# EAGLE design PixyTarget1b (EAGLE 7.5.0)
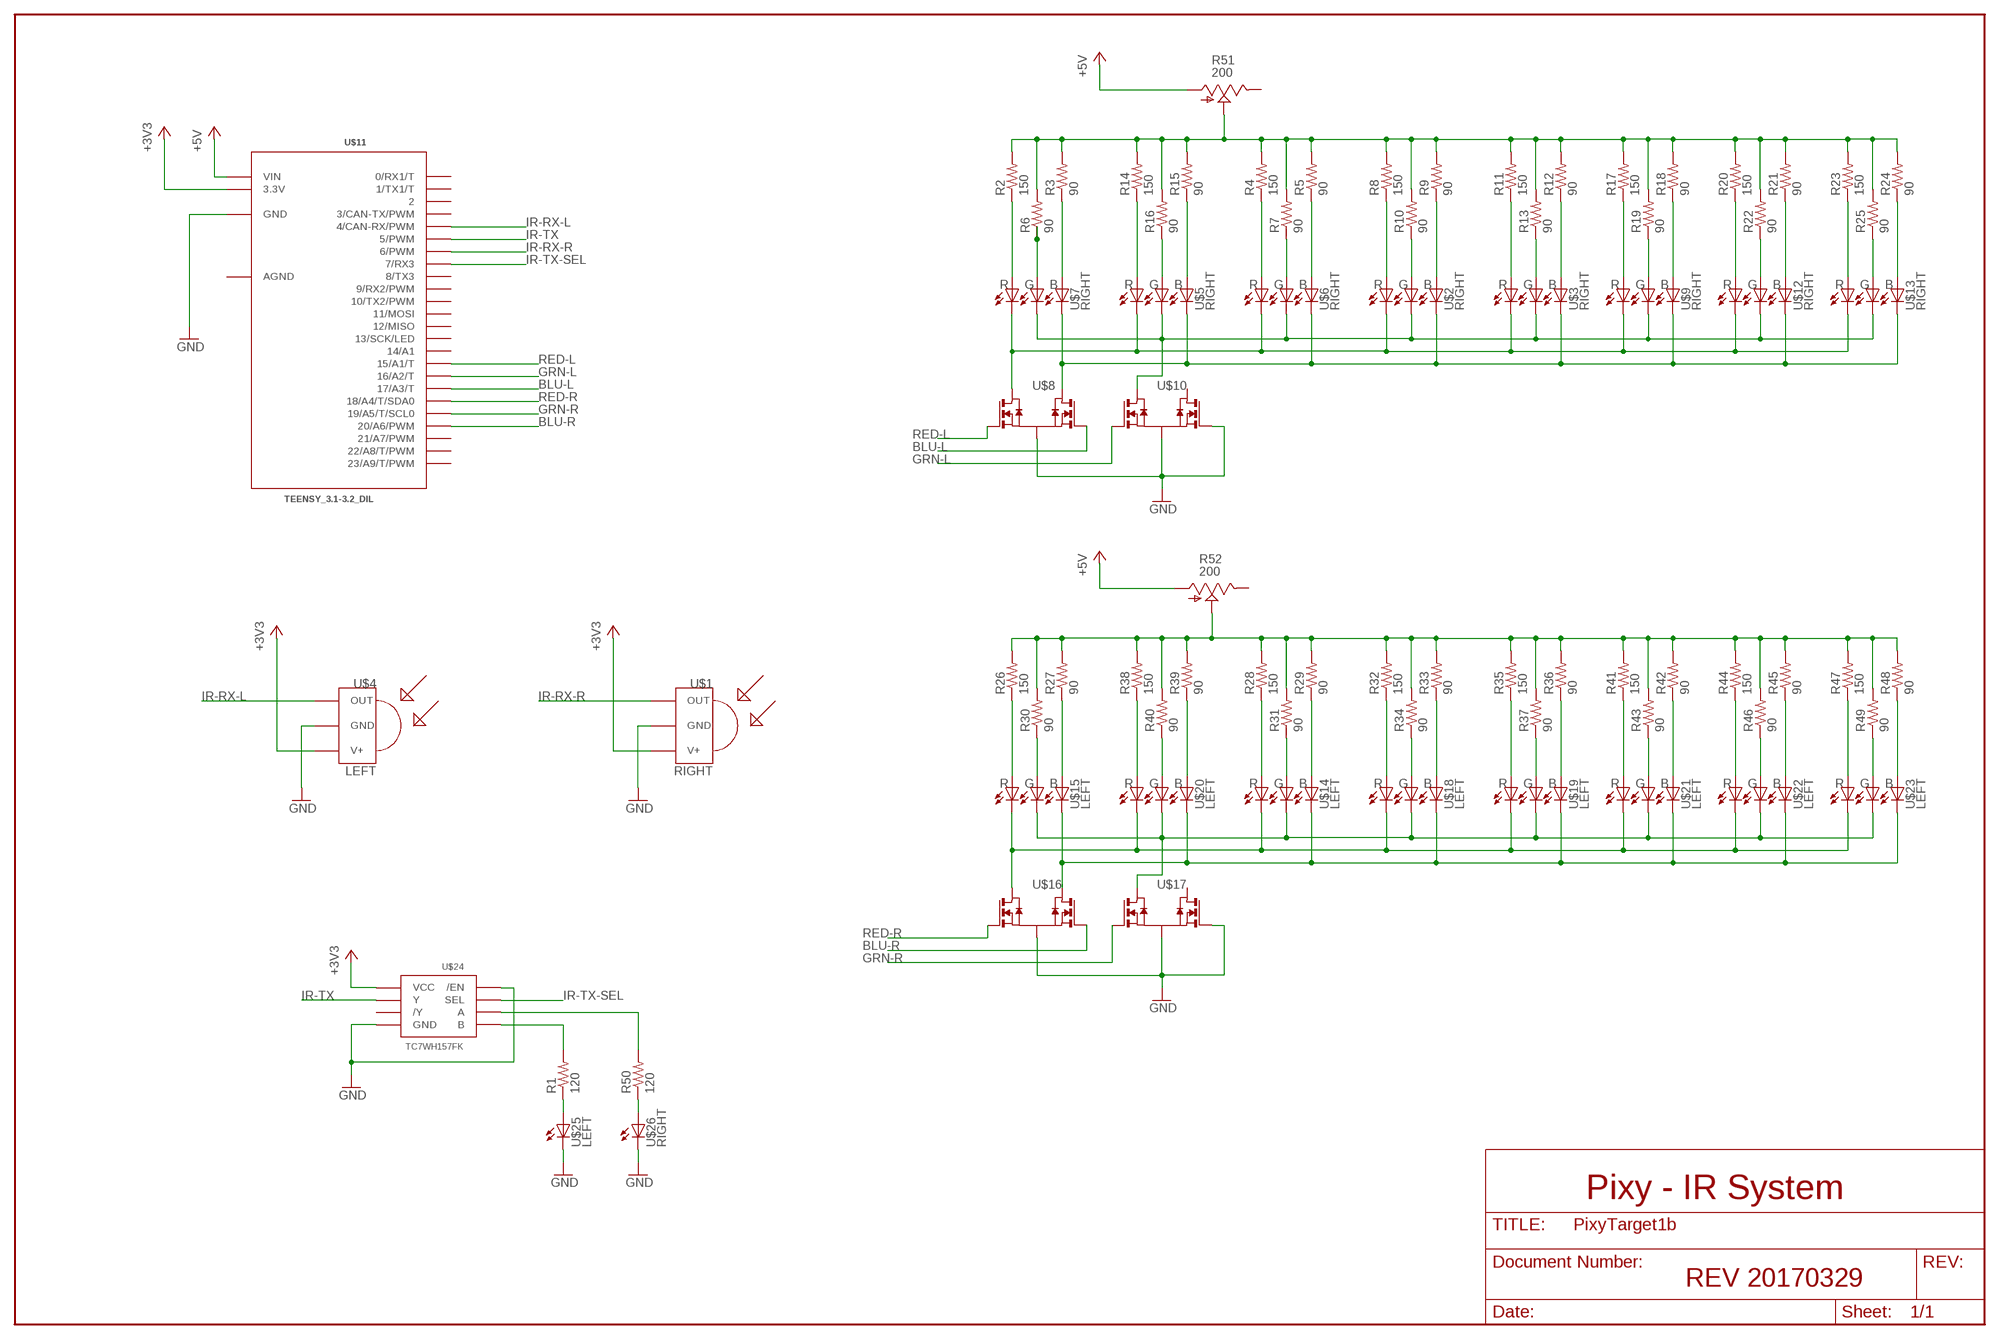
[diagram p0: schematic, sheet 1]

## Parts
R1  120  R-US_R1206  [R1206]
R2  150  R-US_R1206  [R1206]
R3  90  R-US_R1206  [R1206]
R4  150  R-US_R1206  [R1206]
R5  90  R-US_R1206  [R1206]
R6  90  R-US_R1206  [R1206]
R7  90  R-US_R1206  [R1206]
R8  150  R-US_R1206  [R1206]
R9  90  R-US_R1206  [R1206]
R10  90  R-US_R1206  [R1206]
R11  150  R-US_R1206  [R1206]
R12  90  R-US_R1206  [R1206]
R13  90  R-US_R1206  [R1206]
R14  150  R-US_R1206  [R1206]
R15  90  R-US_R1206  [R1206]
R16  90  R-US_R1206  [R1206]
R17  150  R-US_R1206  [R1206]
R18  90  R-US_R1206  [R1206]
R19  90  R-US_R1206  [R1206]
R20  150  R-US_R1206  [R1206]
R21  90  R-US_R1206  [R1206]
R22  90  R-US_R1206  [R1206]
R23  150  R-US_R1206  [R1206]
R24  90  R-US_R1206  [R1206]
R25  90  R-US_R1206  [R1206]
R26  150  R-US_R1206  [R1206]
R27  90  R-US_R1206  [R1206]
R28  150  R-US_R1206  [R1206]
R29  90  R-US_R1206  [R1206]
R30  90  R-US_R1206  [R1206]
R31  90  R-US_R1206  [R1206]
R32  150  R-US_R1206  [R1206]
R33  90  R-US_R1206  [R1206]
R34  90  R-US_R1206  [R1206]
R35  150  R-US_R1206  [R1206]
R36  90  R-US_R1206  [R1206]
R37  90  R-US_R1206  [R1206]
R38  150  R-US_R1206  [R1206]
R39  90  R-US_R1206  [R1206]
R40  90  R-US_R1206  [R1206]
R41  150  R-US_R1206  [R1206]
R42  90  R-US_R1206  [R1206]
R43  90  R-US_R1206  [R1206]
R44  150  R-US_R1206  [R1206]
R45  90  R-US_R1206  [R1206]
R46  90  R-US_R1206  [R1206]
R47  150  R-US_R1206  [R1206]
R48  90  R-US_R1206  [R1206]
R49  90  R-US_R1206  [R1206]
R50  120  R-US_R1206  [R1206]
R51  200  TRIM_US-B25P  [B25P]
R52  200  TRIM_US-B25P  [B25P]
U$1  RIGHT  TSOP3X  [TSOP18XX]
U$2  RIGHT  LED_RGB_6SMD  [6-PLCC]
U$3  RIGHT  LED_RGB_6SMD  [6-PLCC]
U$4  LEFT  TSOP3X  [TSOP18XX]
U$5  RIGHT  LED_RGB_6SMD  [6-PLCC]
U$6  RIGHT  LED_RGB_6SMD  [6-PLCC]
U$7  RIGHT  LED_RGB_6SMD  [6-PLCC]
U$8  QS5K2TR  [SOT-23-5]
U$9  RIGHT  LED_RGB_6SMD  [6-PLCC]
U$10  QS5K2TR  [SOT-23-5]
U$11  TEENSY_3.1-3.2_DIL  [TEENSY_3.0-3.2&LC_DIL]
U$12  RIGHT  LED_RGB_6SMD  [6-PLCC]
U$13  RIGHT  LED_RGB_6SMD  [6-PLCC]
U$14  LEFT  LED_RGB_6SMD  [6-PLCC]
U$15  LEFT  LED_RGB_6SMD  [6-PLCC]
U$16  QS5K2TR  [SOT-23-5]
U$17  QS5K2TR  [SOT-23-5]
U$18  LEFT  LED_RGB_6SMD  [6-PLCC]
U$19  LEFT  LED_RGB_6SMD  [6-PLCC]
U$20  LEFT  LED_RGB_6SMD  [6-PLCC]
U$21  LEFT  LED_RGB_6SMD  [6-PLCC]
U$22  LEFT  LED_RGB_6SMD  [6-PLCC]
U$23  LEFT  LED_RGB_6SMD  [6-PLCC]
U$24  TC7WH157FK  [SSOP8-P-0.65]
U$25  LEFT  LED5MM  [LED5MM]
U$26  RIGHT  LED5MM  [LED5MM]

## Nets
+3V3: U$1.VCC(V+) U$4.VCC(V+) U$11.3.3V U$24.P$8(VCC)
+5V: R51.A R52.A U$11.VIN
BLU-L: U$8.3(G2) U$11.17/A3(17/A3/T)
BLU-R: U$11.20/A6(20/A6/PWM) U$16.3(G2)
GND [ground]: U$1.GND U$4.GND U$8.2(S) U$10.2(S) U$10.3(G2) U$11.GND U$16.2(S) U$17.2(S) U$17.3(G2) U$24.P$4(GND) U$24.P$7(/EN) U$25.K(C) U$26.K(C)
GRN-L: U$10.1(G1) U$11.16/A2(16/A2/T)
GRN-R: U$11.19/A5(19/A5/T/SCL0) U$17.1(G1)
IR-RX-L: U$4.OUT U$11.4(4/CAN-RX/PWM)
IR-RX-R: U$1.OUT U$11.6(6/PWM)
IR-TX: U$11.5(5/PWM) U$24.P$5(Y)
IR-TX-SEL: U$11.7(7/RX3) U$24.P$6(SEL)
N$1: R8.1 U$2.P$1(A1)
N$2: R9.1 U$2.P$3(A3)
N$3: R2.1 U$7.P$1(A1)
N$4: R3.1 U$7.P$3(A3)
N$5: R6.1 U$7.P$2(A2)
N$6: R26.1 U$15.P$1(A1)
N$7: R10.1 U$2.P$2(A2)
N$8: U$2.P$6(C1) U$3.P$6(C1) U$5.P$6(C1) U$6.P$6(C1) U$7.P$6(C1) U$8.5(D1) U$9.P$6(C1) U$12.P$6(C1) U$13.P$6(C1)
N$9: U$2.P$4(C3) U$3.P$4(C3) U$5.P$4(C3) U$6.P$4(C3) U$7.P$4(C3) U$8.4(D2) U$9.P$4(C3) U$12.P$4(C3) U$13.P$4(C3)
N$10: R1.1 U$25.A
N$11: R20.1 U$12.P$1(A1)
N$12: R11.1 U$3.P$1(A1)
N$13: R12.1 U$3.P$3(A3)
N$14: R13.1 U$3.P$2(A2)
N$15: R17.1 U$9.P$1(A1)
N$16: R18.1 U$9.P$3(A3)
N$17: R14.1 U$5.P$1(A1)
N$18: R15.1 U$5.P$3(A3)
N$19: R19.1 U$9.P$2(A2)
N$20: R21.1 U$12.P$3(A3)
N$21: R16.1 U$5.P$2(A2)
N$22: U$2.P$5(C2) U$3.P$5(C2) U$5.P$5(C2) U$6.P$5(C2) U$7.P$5(C2) U$9.P$5(C2) U$10.5(D1) U$12.P$5(C2) U$13.P$5(C2)
N$23: R22.1 U$12.P$2(A2)
N$24: R27.1 U$15.P$3(A3)
N$25: R4.1 U$6.P$1(A1)
N$26: R5.1 U$6.P$3(A3)
N$27: R30.1 U$15.P$2(A2)
N$28: R7.1 U$6.P$2(A2)
N$29: R23.1 U$13.P$1(A1)
N$30: R24.1 U$13.P$3(A3)
N$31: R25.1 U$13.P$2(A2)
N$32: R28.1 U$14.P$1(A1)
N$33: R29.1 U$14.P$3(A3)
N$34: R31.1 U$14.P$2(A2)
N$35: R32.1 U$18.P$1(A1)
N$36: R33.1 U$18.P$3(A3)
N$37: R34.1 U$18.P$2(A2)
N$38: U$14.P$6(C1) U$15.P$6(C1) U$16.5(D1) U$18.P$6(C1) U$19.P$6(C1) U$20.P$6(C1) U$21.P$6(C1) U$22.P$6(C1) U$23.P$6(C1)
N$39: R35.1 U$19.P$1(A1)
N$40: R36.1 U$19.P$3(A3)
N$41: R37.1 U$19.P$2(A2)
N$42: U$14.P$4(C3) U$15.P$4(C3) U$16.4(D2) U$18.P$4(C3) U$19.P$4(C3) U$20.P$4(C3) U$21.P$4(C3) U$22.P$4(C3) U$23.P$4(C3)
N$43: R38.1 U$20.P$1(A1)
N$44: R39.1 U$20.P$3(A3)
N$45: R40.1 U$20.P$2(A2)
N$46: U$14.P$5(C2) U$15.P$5(C2) U$17.5(D1) U$18.P$5(C2) U$19.P$5(C2) U$20.P$5(C2) U$21.P$5(C2) U$22.P$5(C2) U$23.P$5(C2)
N$47: R41.1 U$21.P$1(A1)
N$48: R42.1 U$21.P$3(A3)
N$49: R43.1 U$21.P$2(A2)
N$50: R44.1 U$22.P$1(A1)
N$51: R45.1 U$22.P$3(A3)
N$52: R46.1 U$22.P$2(A2)
N$53: R47.1 U$23.P$1(A1)
N$54: R48.1 U$23.P$3(A3)
N$55: R49.1 U$23.P$2(A2)
N$56: R50.2 U$24.P$1(A)
N$57: R50.1 U$26.A
N$58: R1.2 U$24.P$2(B)
N$59: R2.2 R3.2 R4.2 R5.2 R6.2 R7.2 R8.2 R9.2 R10.2 R11.2 R12.2 R13.2 R14.2 R15.2 R16.2 R17.2 R18.2 R19.2 R20.2 R21.2 R22.2 R23.2 R24.2 R25.2 R51.S
N$60: R26.2 R27.2 R28.2 R29.2 R30.2 R31.2 R32.2 R33.2 R34.2 R35.2 R36.2 R37.2 R38.2 R39.2 R40.2 R41.2 R42.2 R43.2 R44.2 R45.2 R46.2 R47.2 R48.2 R49.2 R52.S
RED-L: U$8.1(G1) U$11.15/A1(15/A1/T)
RED-R: U$11.18/A4(18/A4/T/SDA0) U$16.1(G1)
Unconnected: R51.E R52.E U$10.4(D2) U$11.0(0/RX1/T) U$11.1(1/TX1/T) U$11.2 U$11.3(3/CAN-TX/PWM) U$11.8(8/TX3) U$11.9(9/RX2/PWM) U$11.10(10/TX2/PWM) U$11.11(11/MOSI) U$11.12(12/MISO) U$11.13(13/SCK/LED) U$11.14/A0(14/A1) U$11.21/A7(21/A7/PWM) U$11.22/A8(22/A8/T/PWM) U$11.23/A9(23/A9/T/PWM) U$17.4(D2) U$24.P$3(/Y)

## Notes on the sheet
- Pixy - IR System
- REV 20170329

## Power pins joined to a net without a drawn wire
GND: U$11.AGND

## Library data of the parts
R1-R50 = resistor:R-US_: RESISTOR, American symbol
R51 R52 = pot:TRIM_US-: POTENTIOMETER
U$1 U$4 = _Loper:TSOP3X: IR Receiver and Demodulator
U$2 U$3 U$5-U$7 U$9 U$12-U$15 U$18-U$23 = _Loper:LED_RGB_6SMD
U$8 U$10 U$16 U$17 = _Loper:QS5K2TR: MOSFET 2N-CH
U$11 = Teensy_3_and_LC_Series_Boards_v1.4:TEENSY_3.1-3.2_DIL: Teensy 3.1 or 3.2 in a DIL Layout.
U$24 = _Loper:TC7WH157FK: multiplexer 1x 2:1
U$25 U$26 = led:LED: LED

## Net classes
0 default: width 0.406 mm
1 ground: width 0.61 mm

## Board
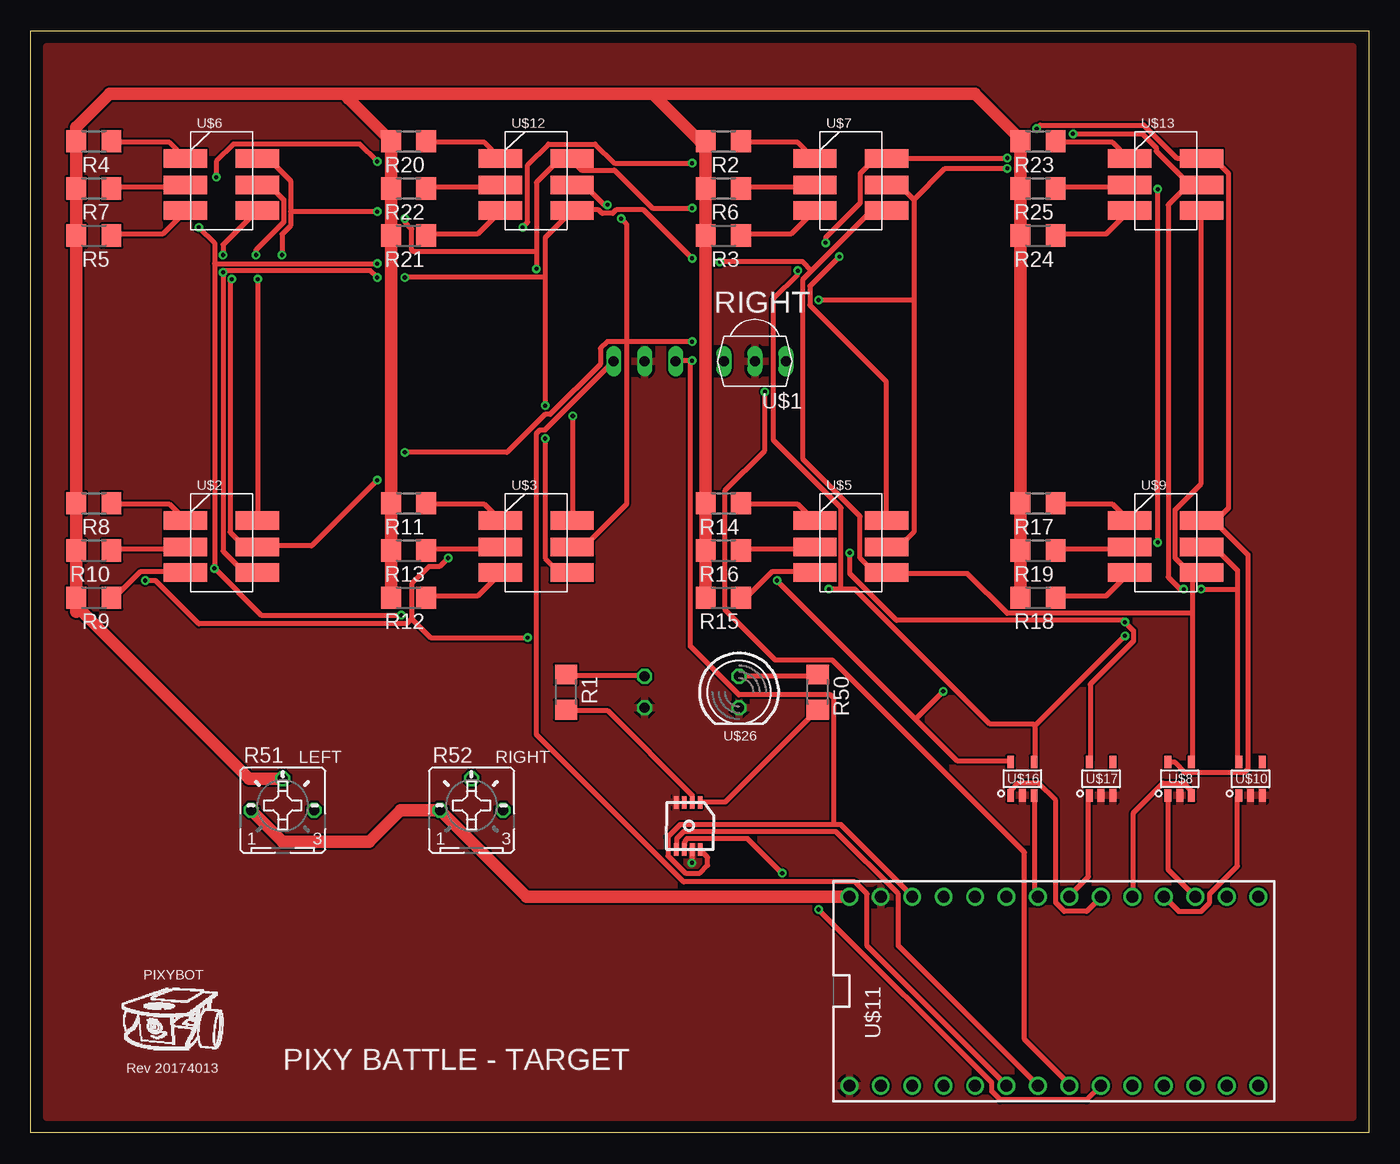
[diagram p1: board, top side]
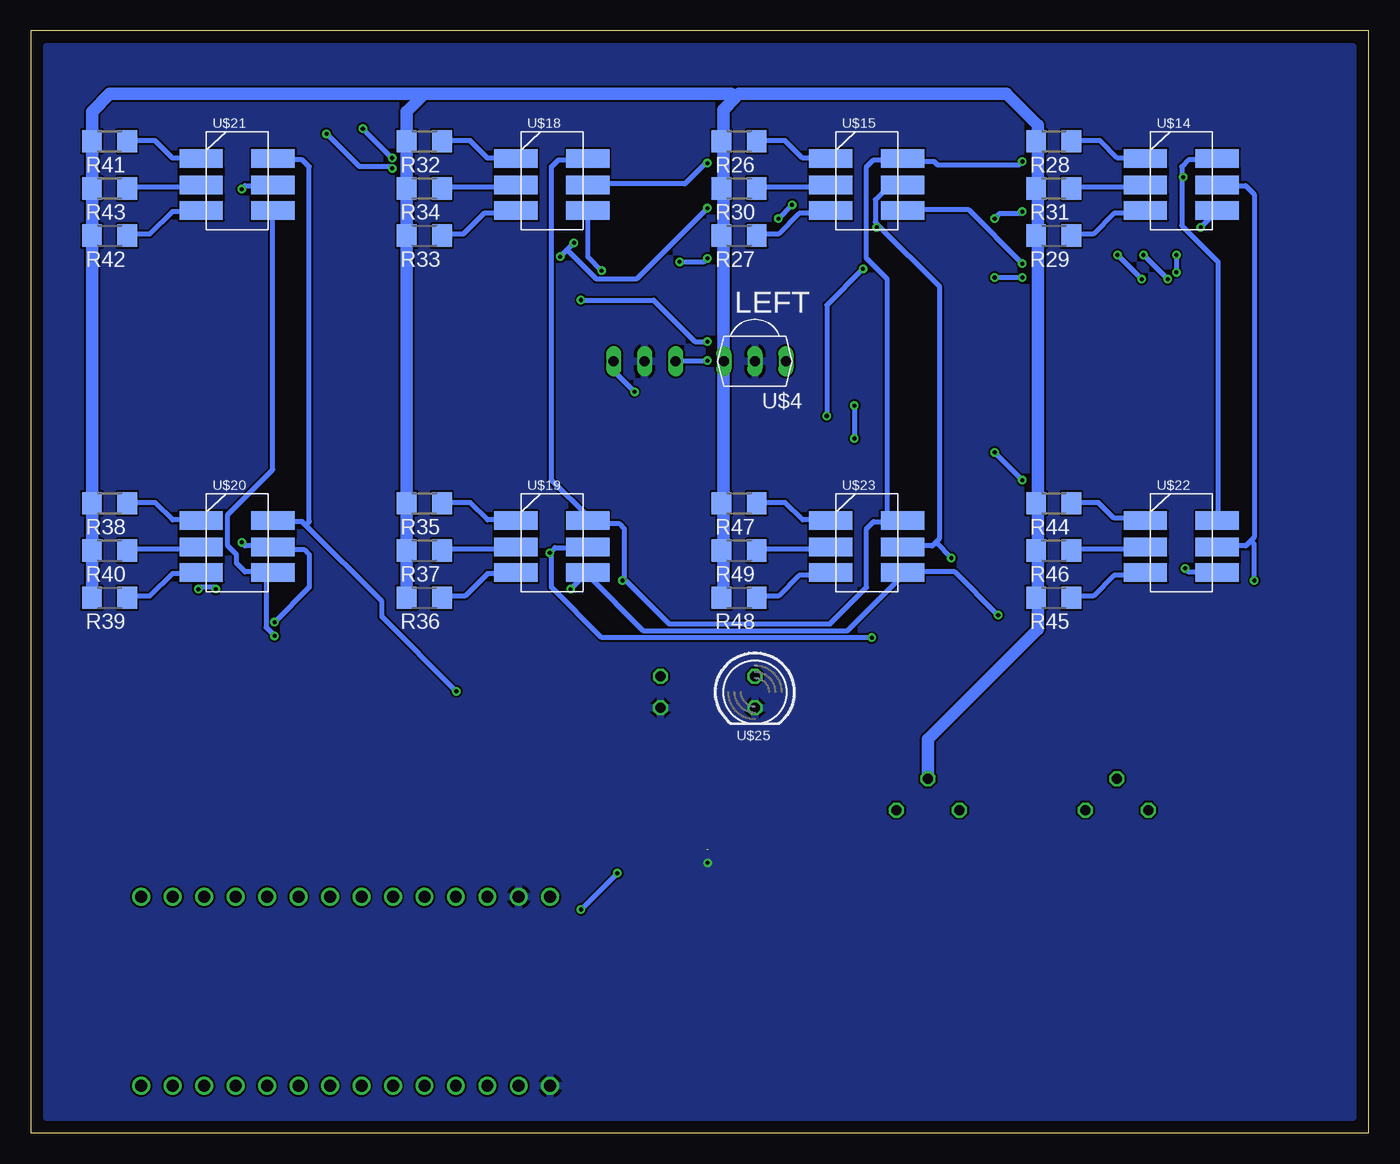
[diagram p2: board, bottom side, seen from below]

Size 107.95 x 88.9 mm. Coordinates in mm from the lower left corner, seen from the top.
Outline: 0,0 0,88.9 107.95,88.9 107.95,0 0,0
Copper layers (1*16): Top 0.0356mm / dielectric 1.5011mm / Bottom 0.0356mm
Design rules "oshpark-2layer": minimum track width 6mil, minimum drill 13mil, track to track 6mil, track to pad 6mil, pad to pad 6mil, via to via 6mil, smd to smd 6mil, copper to edge 15mil, drill to drill 6mil, minimum pad ring 7mil, minimum via ring 7mil, stop-mask expansion 2.5mil, vias tented up to drill 0mil, thermal gap 10mil

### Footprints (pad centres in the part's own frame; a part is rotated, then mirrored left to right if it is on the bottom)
R1206 = smd 1.6 x 1.803: 1 -1.422,0; 2 1.422,0
B25P = drill 0.813 octagon: A -2.54,0; E 2.54,0; S 0,2.54
TSOP18XX = drill 0.813 long: GND -0.001,-0.027; OUT -2.501,-0.027; VCC 2.499,-0.027
6-PLCC = smd 3.5 x 1.5: P$1 -2.77,2.41; P$2 -2.77,0.29; P$3 -2.77,-1.78; P$4 3.03,-1.78; P$5 3.03,0.29; P$6 3.03,2.41
SOT-23-5 = smd 1 x 0.55: 1 -1.35,0.95; 2 -1.35,0; 3 -1.35,-0.95; 4 1.35,-0.95; 5 1.35,0.95
TEENSY_3.0-3.2&LC_DIL = drill 0.965: 0 -7.62,13.97; 1 -7.62,11.43; 2 -7.62,8.89; 3 -7.62,6.35; 3.3V 7.62,11.43; 4 -7.62,3.81; 5 -7.62,1.27; 6 -7.62,-1.27; 7 -7.62,-3.81; 8 -7.62,-6.35; 9 -7.62,-8.89; 10 -7.62,-11.43; 11 -7.62,-13.97; 12 -7.62,-16.51; 13 7.62,-16.51; 14/A0 7.62,-13.97; 15/A1 7.62,-11.43; 16/A2 7.62,-8.89; 17/A3 7.62,-6.35; 18/A4 7.62,-3.81; 19/A5 7.62,-1.27; 20/A6 7.62,1.27; 21/A7 7.62,3.81; 22/A8 7.62,6.35; 23/A9 7.62,8.89; AGND 7.62,13.97; GND -7.62,16.51; VIN 7.62,16.51
SSOP8-P-0.65 = smd 1 x 0.35: P$1 0,1.95; P$2 0,1.3; P$3 0,0.65; P$4 0,0; P$5 3.8,0; P$6 3.8,0.65; P$7 3.8,1.3; P$8 3.8,1.95
LED5MM = drill 0.813 octagon: A -1.27,0; K 1.27,0

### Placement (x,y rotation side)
R1  43.18,35.56 270 top
R2  55.88,80.01 180 top
R3  55.88,72.39 180 top
R4  5.08,80.01 180 top
R5  5.08,72.39 180 top
R6  55.88,76.2 180 top
R7  5.08,76.2 180 top
R8  5.08,50.8 180 top
R9  5.08,43.18 180 top
R10  5.08,46.99 180 top
R11  30.48,50.8 180 top
R12  30.48,43.18 180 top
R13  30.48,46.99 180 top
R14  55.88,50.8 180 top
R15  55.88,43.18 180 top
R16  55.88,46.99 180 top
R17  81.28,50.8 180 top
R18  81.28,43.18 180 top
R19  81.28,46.99 180 top
R20  30.48,80.01 180 top
R21  30.48,72.39 180 top
R22  30.48,76.2 180 top
R23  81.28,80.01 180 top
R24  81.28,72.39 180 top
R25  81.28,76.2 180 top
R26  50.8,80.01 180 bottom
R27  50.8,72.39 180 bottom
R28  25.4,80.01 180 bottom
R29  25.4,72.39 180 bottom
R30  50.8,76.2 180 bottom
R31  25.4,76.2 180 bottom
R32  76.2,80.01 180 bottom
R33  76.2,72.39 180 bottom
R34  76.2,76.2 180 bottom
R35  76.2,50.8 180 bottom
R36  76.2,43.18 180 bottom
R37  76.2,46.99 180 bottom
R38  101.6,50.8 180 bottom
R39  101.6,43.18 180 bottom
R40  101.6,46.99 180 bottom
R41  101.6,80.01 180 bottom
R42  101.6,72.39 180 bottom
R43  101.6,76.2 180 bottom
R44  25.4,50.8 180 bottom
R45  25.4,43.18 180 bottom
R46  25.4,46.99 180 bottom
R47  50.8,50.8 180 bottom
R48  50.8,43.18 180 bottom
R49  50.8,46.99 180 bottom
R50  63.5,35.56 270 top
R51  20.32,26.04 0 top
R52  35.56,26.04 0 top
U$1  58.42,62.23 180 top
U$2  15.24,46.99 0 top
U$3  40.64,46.99 0 top
U$4  49.53,62.23 180 bottom
U$5  66.04,46.99 0 top
U$6  15.24,76.2 0 top
U$7  66.04,76.2 0 top
U$8  92.71,28.57 90 top
U$9  91.44,46.99 0 top
U$10  98.42,28.57 90 top
U$11  82.55,11.43 90 top
U$12  40.64,76.2 0 top
U$13  91.44,76.2 0 top
U$14  15.24,76.2 0 bottom
U$15  40.64,76.2 0 bottom
U$16  80.01,28.57 90 top
U$17  86.36,28.57 90 top
U$18  66.04,76.2 0 bottom
U$19  66.04,46.99 0 bottom
U$20  91.44,46.99 0 bottom
U$21  91.44,76.2 0 bottom
U$22  15.24,46.99 0 bottom
U$23  40.64,46.99 0 bottom
U$24  52.07,26.67 270 top
U$25  49.53,35.56 270 bottom
U$26  57.15,35.56 270 top

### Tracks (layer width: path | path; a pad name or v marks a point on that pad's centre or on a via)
+3V3  (via drill 0.33)
  Top 0.406: U$4.VCC 52.11,62.31 v53.37,62.31 53.23,62.17 53.23,39.26 57.14,35.34 64.54,35.34 64.82,35.06 64.82,24.87 | 64.82,24.87 65.38,24.87 71.11,19.14 U$11.3.3V | 64.82,24.87 52.39,24.87 51.41,23.89 51.41,22.35 52.81,20.95 53.98,20.95 54.61,21.59 54.61,22.23 54.02,22.82 U$24.P$8
  Bottom 0.406: v53.37,62.31 55.88,62.31 U$1.VCC
+5V
  Top 1.016: U$11.VIN 40.01,19.05 R52.A 29.84,26.04 27.3,23.5 20.32,23.5 R51.A
BLU-L
  Top 0.406: U$8.3 93.6,27.24 93.6,27.66 93.04,28.22 91.36,28.22 88.99,25.84 88.99,19.14 U$11.17/A3
BLU-R
  Top 0.406: U$16.3 81.03,27.1 81.03,19.28 81.17,19.14 U$11.20/A6
GND  (via drill 0.33)  (1 unrouted)
  Top 0.406: 53.34,22.84 v53.34,21.79
  pour Bottom: 1.27,1.27 106.68,1.27 106.68,87.63 1.27,87.63
  pour Top: 1.27,1.27 106.68,1.27 106.68,87.63 1.27,87.63
GRN-L
  Top 0.406: U$10.1 97.37,27.1 97.37,21.51 95.14,19.28 95.14,18.58 94.44,17.88 92.62,17.88 91.5,19 U$11.16/A2
GRN-R
  Top 0.406: U$17.1 85.36,27.1 85.36,20.68 83.82,19.14 U$11.19/A5
IR-RX-L
  Top 0.406: U$4.OUT 46.94,62.17 41.49,56.72 41.07,56.72 40.79,56.44 40.79,32.13 52.67,20.26 66.5,20.26 67.47,19.28 67.47,15.09 78.65,3.91 U$11.4
IR-RX-R  (via drill 0.33)
  Top 0.406: v59.23,59.79 59.23,55.04 56.02,51.83 56.02,42.19 60.07,38.14 64.68,38.14 80.19,22.63 80.19,7.54 83.82,3.91 U$11.6
  Bottom 0.406: v59.23,59.79 60.91,61.47 60.91,62.17 U$1.OUT
IR-TX
  Top 0.406: U$24.P$5 52.11,22.91 52.11,23.75 52.67,24.31 64.96,24.31 69.99,19.28 69.99,15.09 81.17,3.91 U$11.5
IR-TX-SEL  (via drill 0.33)
  Top 0.406: v60.63,20.95 57.84,23.75 52.95,23.75 52.81,23.61 52.73,23.42 U$24.P$6 | v63.56,18.02 77.53,4.05 77.53,3.35 78.23,2.65 85.22,2.65 86.33,3.77 U$11.7
  Bottom 0.406: v63.56,18.02 v60.63,20.95
N$1
  Top 0.406: R8.1 6.57,50.71 11.18,50.71 12.43,49.45 U$2.P$1
N$2
  Top 0.406: R9.1 6.57,43.31 6.84,43.31 8.8,45.26 12.43,45.26 U$2.P$3
N$3
  Top 0.406: R2.1 57.42,79.91 61.89,79.91 63.14,78.65 U$7.P$1
N$4
  Top 0.406: R3.1 57.42,72.5 61.33,72.5 63.14,74.32 U$7.P$3
N$5
  Top 0.406: R6.1 57.42,76.28 63.01,76.28 63.14,76.42 U$7.P$2
N$6
  Bottom 0.406: R26.1 49.31,80.05 47.08,80.05 45.68,78.65 43.45,78.65 U$15.P$1
N$7
  Top 0.406: R10.1 6.57,47.08 12.29,47.08 12.43,47.22 U$2.P$2
N$8  (via drill 0.33)
  Top 0.406: U$8.5 91.78,29.9 92.34,29.9 93.18,29.06 97.93,29.06 98.21,29.34 98.21,46.66 95.56,49.31 94.58,49.31 U$9.P$6 95.69,49.45 96.67,50.43 96.67,77.39 95.56,78.51 94.58,78.51 U$13.P$6 94.3,78.65 92.48,78.65 89.83,81.31 81.44,81.31 v81.17,81.03 | v65.24,70.69 62.87,68.31 62.87,66.78 69.01,60.63 69.01,49.45 U$5.P$6 | v64.12,71.81 64.12,72.22 66.92,75.02 66.92,77.39 68.03,78.51 69.01,78.51 U$7.P$6 69.15,78.65 v78.79,78.65 | v18.3,68.87 18.3,49.45 U$2.P$6 | v20.26,70.83 20.26,72.5 20.95,73.2 20.95,74.32 | 20.95,74.32 20.95,76.83 19.28,78.51 18.3,78.51 U$6.P$6 | v43.73,57.84 43.73,49.45 U$3.P$6 | 40.79,71.11 40.79,76.69 42.61,78.51 43.59,78.51 U$12.P$6 43.73,78.37 44.42,77.67 47.08,77.67 50.15,74.6 v53.37,74.6 | 40.79,71.11 v40.79,69.71 | v27.94,74.32 20.95,74.32 | v30.18,73.76 30.18,73.48 30.73,72.92 30.73,71.25 30.87,71.11 40.79,71.11
  Bottom 0.406: v64.12,71.81 64.68,71.25 | 64.68,71.25 v65.24,70.69 | v20.26,70.83 v18.3,68.87 | v43.73,57.84 43.73,66.78 v40.79,69.71 | v27.94,74.32 28.08,74.18 29.76,74.18 v30.18,73.76 | 64.68,71.25 62.31,68.87 59.09,68.87 v53.37,74.6 | v78.79,78.65 v81.17,81.03
N$9  (via drill 0.33)
  Top 0.406: v15.51,70.83 15.51,71.67 18.16,74.32 U$6.P$4 | U$2.P$4 18.16,45.26 17.18,45.26 15.51,46.94 v15.51,69.43 15.65,69.57 27.38,69.57 v27.94,69.01 | v41.49,56.02 41.49,46.38 42.61,45.26 43.59,45.26 U$3.P$4 | 41.49,69.01 41.49,72.22 43.59,74.32 U$12.P$4 43.87,74.46 45.82,74.46 46.1,74.18 46.94,74.18 47.22,74.46 49.45,74.46 v53.37,70.55 | 41.49,69.01 v41.49,58.67 | 93.74,41.91 93.74,44.42 94.44,45.12 U$9.P$4 93.88,44.84 92.34,46.38 92.34,50.29 94.44,52.39 94.44,74.32 U$13.P$4 | 93.74,41.91 93.74,30.04 U$8.4 | 93.74,41.91 78.79,41.91 75.58,45.12 69.15,45.12 U$5.P$4 68.87,45.26 68.03,45.26 66.92,46.38 66.92,49.73 62.31,54.34 62.31,68.87 63.01,69.57 | 63.01,69.57 67.75,74.32 69.01,74.32 U$7.P$4 | v55.6,70.27 62.31,70.27 63.01,69.57 | 41.49,69.01 v30.18,69.01
  Bottom 0.406: v15.51,70.83 v15.51,69.43 | v41.49,58.67 v41.49,56.02 | v53.37,70.55 53.65,70.27 v55.6,70.27 | v30.18,69.01 v27.94,69.01
N$10
  Top 0.406: R1.1 43.31,36.88 49.45,36.88 U$25.A
N$11
  Top 0.406: R20.1 31.99,79.91 36.6,79.91 37.86,78.65 U$12.P$1
N$12
  Top 0.406: R11.1 31.99,50.71 36.6,50.71 37.86,49.45 U$3.P$1
N$13
  Top 0.406: R12.1 31.99,43.31 36.04,43.31 37.86,45.12 U$3.P$3
N$14
  Top 0.406: R13.1 31.99,47.08 37.72,47.08 37.86,47.22 U$3.P$2
N$15
  Top 0.406: R17.1 82.7,50.71 87.31,50.71 88.57,49.45 U$9.P$1
N$16
  Top 0.406: R18.1 82.7,43.31 86.75,43.31 88.57,45.12 U$9.P$3
N$17
  Top 0.406: R14.1 57.42,50.71 61.89,50.71 63.14,49.45 U$5.P$1
N$18
  Top 0.406: R15.1 57.42,43.31 57.84,43.31 59.79,45.26 63.14,45.26 U$5.P$3
N$19
  Top 0.406: R19.1 82.7,47.08 88.43,47.08 88.57,47.22 U$9.P$2
N$20
  Top 0.406: R21.1 31.99,72.5 36.04,72.5 37.86,74.32 U$12.P$3
N$21
  Top 0.406: R16.1 57.42,47.08 63.01,47.08 63.14,47.22 U$5.P$2
N$22  (via drill 0.33)
  Top 0.406: v16.2,68.87 16.07,68.73 16.07,48.48 17.18,47.36 18.16,47.36 U$2.P$5 18.44,47.36 22.63,47.36 v27.94,52.67 | v18.16,70.83 18.16,71.25 20.4,73.48 20.4,75.3 19.28,76.42 18.3,76.42 U$6.P$5 | 48.06,63.84 48.06,73.34 v47.64,73.76 | 48.06,63.84 48.06,50.71 44.7,47.36 43.73,47.36 U$3.P$5 | v46.52,74.88 46.24,74.88 44.7,76.42 43.73,76.42 U$12.P$5 | v30.18,54.9 38.42,54.9 41.49,57.98 41.91,57.98 45.96,62.03 45.96,63.28 46.52,63.84 48.06,63.84 | 97.37,43.87 97.37,45.4 95.56,47.22 94.58,47.22 U$9.P$5 | 97.37,43.87 97.37,30.04 U$10.5 | 71.25,75.3 71.25,67.2 | 71.25,67.2 71.25,48.48 70.13,47.36 69.15,47.36 U$5.P$5 | 71.25,75.3 70.13,76.42 69.15,76.42 U$7.P$5 | v84.1,80.61 89.69,80.61 90.81,79.49 90.81,79.21 93.46,76.56 94.44,76.56 U$13.P$5 93.32,76.42 91.78,74.88 91.78,44.84 92.76,43.87 v93.04,43.87 | v78.79,77.81 73.76,77.81 71.25,75.3 | v94.44,43.87 97.37,43.87 | v53.37,63.84 48.06,63.84 | 71.25,67.2 v63.56,67.2
  Bottom 0.406: v18.16,70.83 v16.2,68.87 | v46.52,74.88 v47.64,73.76 | v30.18,54.9 v27.94,52.67 | v84.1,80.61 81.44,77.95 78.93,77.95 v78.79,77.81 | v94.44,43.87 94.3,44.01 93.18,44.01 v93.04,43.87 | v53.37,63.84 54.34,63.84 57.7,67.2 v63.56,67.2
N$23
  Top 0.406: R22.1 31.99,76.28 37.72,76.28 37.86,76.42 U$12.P$2
N$24
  Bottom 0.406: R27.1 49.31,72.5 47.64,72.5 45.96,74.18 43.59,74.18 43.45,74.32 U$15.P$3
N$25
  Top 0.406: R4.1 6.57,79.91 11.18,79.91 12.43,78.65 U$6.P$1
N$26
  Top 0.406: R5.1 6.57,72.5 10.62,72.5 12.43,74.32 U$6.P$3
N$27
  Bottom 0.406: R30.1 49.31,76.28 43.59,76.28 43.45,76.42 U$15.P$2
N$28
  Top 0.406: R7.1 6.57,76.28 12.29,76.28 12.43,76.42 U$6.P$2
N$29
  Top 0.406: R23.1 82.7,79.91 87.31,79.91 88.57,78.65 U$13.P$1
N$30
  Top 0.406: R24.1 82.7,72.5 86.75,72.5 88.57,74.32 U$13.P$3
N$31
  Top 0.406: R25.1 82.7,76.28 88.43,76.28 88.57,76.42 U$13.P$2
N$32
  Bottom 0.406: R28.1 23.89,80.05 21.65,80.05 20.26,78.65 18.02,78.65 U$14.P$1
N$33
  Bottom 0.406: R29.1 23.89,72.5 22.21,72.5 20.54,74.18 18.16,74.18 18.02,74.32 U$14.P$3
N$34
  Bottom 0.406: R31.1 23.89,76.28 18.16,76.28 18.02,76.42 U$14.P$2
N$35
  Bottom 0.406: R32.1 74.74,80.05 72.5,80.05 71.11,78.65 68.87,78.65 U$18.P$1
N$36
  Bottom 0.406: R33.1 74.74,72.5 73.06,72.5 71.39,74.18 69.01,74.18 68.87,74.32 U$18.P$3
N$37
  Bottom 0.406: R34.1 74.74,76.28 69.01,76.28 68.87,76.42 U$18.P$2
N$38  (via drill 0.33)
  Top 0.406: v60.21,44.56 71.39,33.39 | 71.39,33.39 74.74,30.04 78.93,30.04 U$16.5 | 71.39,33.39 v73.62,35.62 | v14.95,77.11 14.95,78.37 16.34,79.77 26.54,79.77 v27.94,78.37
  Bottom 0.406: 15.09,77.11 15.09,77.95 14.53,78.51 12.29,78.51 U$14.P$6 | 15.09,77.11 15.09,73.2 12.15,70.27 12.15,49.45 U$22.P$6 | 85.78,49.03 79.63,42.89 79.63,41.63 v73.62,35.62 | 85.78,49.03 86.06,49.31 88.29,49.31 U$20.P$6 | U$18.P$6 63.14,78.51 65.38,78.51 65.94,77.95 65.94,52.67 63.01,49.73 63.01,49.59 U$19.P$6 63.01,49.31 62.87,49.17 60.49,49.17 60.07,48.76 60.07,44.7 v60.21,44.56 59.93,44.56 56.44,41.07 43.45,41.07 40.51,44.01 40.51,48.76 39.95,49.31 37.72,49.31 U$23.P$6 38.84,49.45 38.84,68.87 40.51,70.55 40.51,77.95 39.95,78.51 37.72,78.51 U$15.P$6 37.58,78.37 35.06,78.37 34.78,78.09 28.22,78.09 v27.94,78.37 | U$21.P$6 88.29,78.51 86.06,78.51 85.5,77.95 85.5,49.31 85.78,49.03 | v14.95,77.11 15.09,77.11
N$39
  Bottom 0.406: R35.1 74.74,50.85 72.5,50.85 71.11,49.45 68.87,49.45 U$19.P$1
N$40
  Bottom 0.406: R36.1 74.74,43.31 72.92,43.31 71.11,45.12 68.87,45.12 U$19.P$3
N$41
  Bottom 0.406: R37.1 74.74,47.08 69.01,47.08 68.87,47.22 U$19.P$2
N$42  (via drill 0.33)
  Top 0.406: 14.81,70.13 14.81,71.81 v13.55,73.06 | 14.81,70.13 v14.81,45.54 18.58,41.77 v29.9,41.77 | 14.81,70.13 v27.94,70.13 | 81.03,32.83 81.03,30.04 U$16.4 | v88.29,40.09 81.03,32.83 | 65.38,43.87 66.5,43.87 77.39,32.97 80.89,32.97 81.03,32.83 | 65.38,43.87 v64.4,43.87 | v61.89,69.57 61.89,69.29 59.93,67.33 59.93,55.88 65.38,50.43 65.38,43.87
  Bottom 0.406: v14.81,45.54 14.53,45.26 12.29,45.26 U$22.P$4 | v13.55,73.06 12.29,74.32 U$14.P$4 | v29.9,41.77 33.39,45.26 37.58,45.26 U$23.P$4 37.72,45.12 37.72,44.84 42.05,40.51 58.53,40.51 63.01,44.98 U$19.P$4 63.14,45.12 v64.4,43.87 | v27.94,70.13 32.27,74.46 37.58,74.46 U$15.P$4 | v88.29,40.09 88.99,40.79 88.99,44.56 88.43,45.12 U$20.P$4 89.13,44.7 89.69,45.26 90.67,45.26 91.36,45.96 91.36,46.66 92.06,47.36 92.06,49.87 88.43,53.51 88.43,74.32 U$21.P$4 | v61.89,69.57 63.01,70.69 63.01,74.32 U$18.P$4
N$43
  Bottom 0.406: R38.1 100.17,50.85 97.93,50.85 96.53,49.45 94.3,49.45 U$20.P$1
N$44
  Bottom 0.406: R39.1 100.17,43.31 98.35,43.31 96.53,45.12 94.3,45.12 U$20.P$3
N$45
  Bottom 0.406: R40.1 100.17,47.08 94.44,47.08 94.3,47.22 U$20.P$2
N$46  (via drill 0.33)
  Top 0.406: U$17.5 85.5,30.04 85.5,36.18 88.99,39.67 88.99,40.51 v88.29,41.21 88.15,41.35 69.85,41.35 66.08,45.12 v66.08,46.8 | v90.94,47.64 v90.94,76.14 | v53.37,78.23 47.08,78.23 45.54,79.77 41.77,79.77 40.09,78.09 40.09,73.48 v39.67,73.06 | v9.22,44.56 10.06,44.56 13.55,41.07 30.32,41.07 30.73,41.49 | 30.73,41.49 30.73,44.28 32.13,45.68 32.97,45.68 v33.67,46.38 | v40.09,39.95 32.27,39.95 30.73,41.49
  Bottom 0.406: v88.29,41.21 85.5,44.01 85.5,46.66 85.92,47.08 88.15,47.08 88.29,47.22 U$20.P$5 88.57,47.36 90.67,47.36 v90.94,47.64 | U$19.P$5 63.14,47.22 65.66,47.22 v66.08,46.8 65.94,46.66 65.94,44.01 61.89,39.95 v40.09,39.95 | v90.94,76.14 90.67,76.42 88.43,76.42 U$21.P$5 | 9.5,47.78 9.22,48.06 9.22,75.72 9.92,76.42 12.15,76.42 U$14.P$5 | 9.5,47.78 9.92,47.36 12.15,47.36 U$22.P$5 | 34.92,47.64 34.65,47.92 34.65,68.31 39.53,73.2 | 34.92,47.64 35.2,47.36 37.58,47.36 U$23.P$5 | 39.53,73.2 39.81,73.48 39.81,75.3 38.7,76.42 37.72,76.42 U$15.P$5 | v53.37,78.23 53.51,78.23 55.18,76.56 63.01,76.56 U$18.P$5 | v39.67,73.06 39.53,73.2 | v9.22,44.56 9.22,47.5 9.5,47.78 | 34.92,47.64 v33.67,46.38
N$47
  Bottom 0.406: R41.1 100.17,80.05 97.93,80.05 96.53,78.65 94.3,78.65 U$21.P$1
N$48
  Bottom 0.406: R42.1 100.17,72.5 98.35,72.5 96.53,74.32 94.3,74.32 U$21.P$3
N$49
  Bottom 0.406: R43.1 100.17,76.28 94.44,76.28 94.3,76.42 U$21.P$2
N$50
  Bottom 0.406: R44.1 23.89,50.85 21.79,50.85 20.54,49.59 18.16,49.59 18.02,49.45 U$22.P$1
N$51
  Bottom 0.406: R45.1 23.89,43.31 22.21,43.31 20.54,44.98 18.16,44.98 18.02,45.12 U$22.P$3
N$52
  Bottom 0.406: R46.1 23.89,47.08 18.16,47.08 18.02,47.22 U$22.P$2
N$53
  Bottom 0.406: R47.1 49.31,50.85 47.08,50.85 45.68,49.45 43.45,49.45 U$23.P$1
N$54
  Bottom 0.406: R48.1 49.31,43.31 47.64,43.31 45.96,44.98 43.59,44.98 43.45,45.12 U$23.P$3
N$55
  Bottom 0.406: R49.1 49.31,47.08 43.59,47.08 43.45,47.22 U$23.P$2
N$56
  Top 0.406: U$24.P$1 54.06,26.68 56.02,26.68 63.42,34.09 R50.2
N$57
  Top 0.406: R50.1 63.42,36.88 57.28,36.88 U$26.A
N$58
  Top 0.406: U$24.P$2 53.37,26.68 53.37,27.24 46.52,34.09 43.31,34.09 R1.2
N$59
  Top 0.406: R9.2 3.63,43.31 3.66,43.31 | 3.66,46.94 3.63,46.94 R10.2 | 29.06,47.08 R13.2 | 29.06,47.08 | R5.2 3.63,72.5 3.66,72.5 | 29.06,50.85 R11.2 | 29.06,50.85 | R7.2 3.63,76.28 3.66,76.28 | 29.06,72.5 R21.2 | 29.06,72.5 | R16.2 54.48,47.08 54.46,47.08 | 29.06,76.28 R22.2 | 29.06,76.28 | R14.2 54.48,50.85 54.46,50.85 | R19.2 79.91,47.08 79.86,47.08 | R3.2 54.48,72.5 54.46,72.5 | R17.2 79.91,50.85 79.86,50.85 | R6.2 54.48,76.28 54.46,76.28 | R24.2 79.91,72.5 79.86,72.5 | R25.2 79.91,76.28 79.86,76.28
  Top 1.016: 3.66,42.55 R9.2 3.66,43.31 3.66,46.94 R10.2 R8.2 R5.2 3.66,72.5 R7.2 3.66,76.28 R4.2 3.66,81.13 6.35,83.82 25.25,83.82 25.64,83.43 | 3.66,42.55 3.66,42.06 | R15.2 R16.2 54.46,47.08 R14.2 54.46,50.85 R3.2 54.46,72.5 R6.2 54.46,76.28 R2.2 53.98,80.01 50.16,83.82 | R18.2 R19.2 79.86,47.08 R17.2 79.86,50.85 R24.2 79.86,72.5 R25.2 79.86,76.28 R23.2 79.86,80.16 76.2,83.82 50.16,83.82 | R51.S 17.63,28.57 3.66,42.55 | 25.64,83.43 R20.2 29.06,76.28 R22.2 29.06,72.5 R21.2 29.06,50.85 R11.2 29.06,47.08 R13.2 R12.2 | 50.16,83.82 25.4,83.82 25.64,83.43
N$60
  Bottom 0.406: R45.2 26.82,43.31 26.67,43.31 | 26.67,50.85 26.68,50.85 R44.2 | R46.2 26.82,47.08 26.67,47.08 | R49.2 52.25,47.08 52.07,47.08 | R29.2 26.82,72.5 26.67,72.5 | R47.2 52.25,50.85 52.07,50.85 | R31.2 26.82,76.28 26.67,76.28 | R37.2 77.67,47.08 77.62,47.08 | R27.2 52.25,72.5 52.07,72.5 | R35.2 77.67,50.85 77.62,50.85 | R30.2 52.25,76.28 52.07,76.28 | R26.2 52.25,80.05 52.07,80.05 | R40.2 103.1,47.08 103.02,47.08 | R33.2 77.67,72.5 77.62,72.5 | R38.2 103.1,50.85 103.02,50.85 | R34.2 77.67,76.28 77.62,76.28 | R32.2 77.67,80.05 77.62,80.05 | R42.2 103.1,72.5 103.02,72.5 | R43.2 103.1,76.28 103.02,76.28 | R41.2 103.1,80.05 103.02,80.05
  Bottom 1.016: R52.S 35.56,31.75 26.67,40.64 26.67,43.31 26.67,47.08 26.67,50.85 26.67,72.5 26.67,76.28 26.67,79.86 | 26.67,79.86 R28.2 | 26.67,79.86 26.67,81.28 29.21,83.82 50.8,83.82 51.12,83.5 | 51.12,83.5 52.07,82.55 52.07,80.05 52.07,76.28 52.07,72.5 52.07,50.85 52.07,47.08 52.07,43.33 R48.2 | R36.2 R37.2 77.62,47.08 R35.2 77.62,50.85 R33.2 77.62,72.5 R34.2 77.62,76.28 R32.2 77.62,80.05 77.62,82.4 76.2,83.82 | 76.2,83.82 51.44,83.82 51.12,83.5 | R39.2 R40.2 103.02,47.08 R38.2 103.02,50.85 R42.2 103.02,72.5 R43.2 103.02,76.28 R41.2 103.02,80.05 103.02,82.4 101.6,83.82 76.2,83.82
RED-L
  Top 0.406: U$8.1 91.78,27.1 91.78,21.23 93.88,19.14 U$11.15/A1
RED-R
  Top 0.406: U$16.1 79.07,27.24 79.07,27.66 79.63,28.22 81.31,28.22 82.7,26.82 82.7,18.58 83.4,17.88 85.22,17.88 86.33,19 U$11.18/A4

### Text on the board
tPlace: LEFT | RIGHT | PIXYBOT | Rev 20174013 | PIXY BATTLE - TARGET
